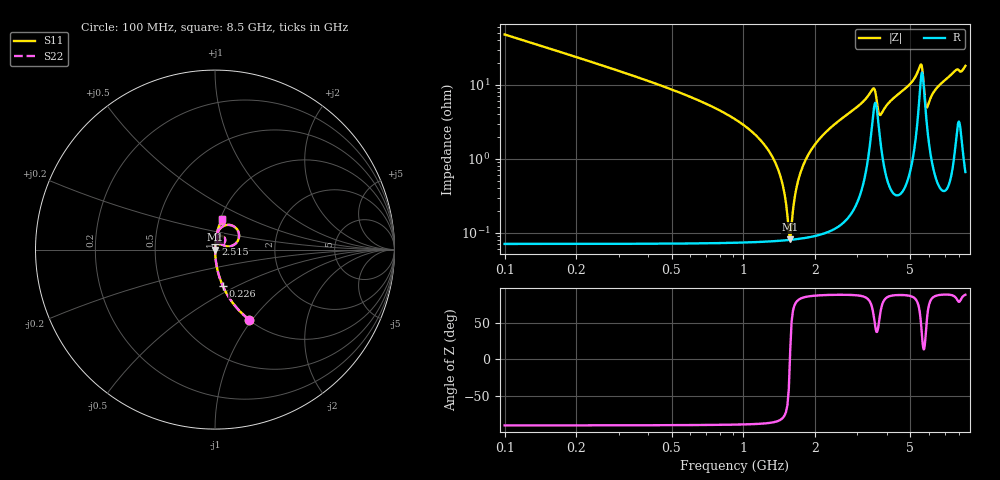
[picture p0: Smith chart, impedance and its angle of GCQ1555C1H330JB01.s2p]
!Murata Part Number: GCQ1555C1H330JB01
!These Parameters are Measured in Series Mode Connection
!Data Generated on Mar 13, 2026
!  o--ll--o
!Port1  Port2
!  o------o
!Operation Temp=25[degC], DC Bias Voltage=0[V]
!Freq. Start=100[MHz] Stop=9[GHz] 401[Steps]
# Hz S RI R 50
!Freq.(Hz) S11(Real) S11(Imag) S21(Real) S21(Imag) S12(Real) S12(Imag) S22(Real) S22(Imag)
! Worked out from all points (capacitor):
!   401 points, 100 MHz to 8.5 GHz, reference 50 ohm
!   read as one part in series: C = 33 pF near 142 MHz
!   lowest |Z| = 82.3 mohm at 1.57 GHz (marker M1)
!   series resonance near 1.566 GHz, so ESL is about 310 pH
!   S11 on the Smith chart (normalised r, x): 100 MHz: 1.00, -0.96; 226 MHz: 1.00, -0.42; 2.515 GHz: 1.00, +0.07; 8.5 GHz: 1.01, +0.36
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1e8  0.1878 -0.3898  0.8122 0.3898  0.8122 0.3898  0.1878 -0.3898
2.26e8  0.0425 -0.2  0.9575 0.2  0.9575 0.2  0.0425 -0.2
4.57e8  0.00996 -0.0957  0.99 0.0957  0.99 0.0957  0.00996 -0.0957
1.234e9  0.000986 -0.015  0.999 0.015  0.999 0.015  0.000986 -0.015
1.402e9  0.000829 -0.00693  0.9992 0.00693  0.9992 0.00693  0.000829 -0.00693
1.507e9  0.000801 -0.00241  0.9992 0.00241  0.9992 0.00241  0.000801 -0.00241
1.57e9  0.000805 0.000168  0.9992 -0.000168  0.9992 -0.000168  0.000805 0.000168
1.696e9  0.000854 0.00506  0.9991 -0.00506  0.9991 -0.00506  0.000854 0.00506
1.843e9  0.000971 0.0104  0.999 -0.0104  0.999 -0.0104  0.000971 0.0104
2.116e9  0.00134 0.0197  0.9987 -0.0197  0.9987 -0.0197  0.00134 0.0197
2.515e9  0.00231 0.0328  0.9977 -0.0328  0.9977 -0.0328  0.00231 0.0328
2.914e9  0.00433 0.0468  0.9957 -0.0468  0.9957 -0.0468  0.00433 0.0468
3.481e9  0.0402 0.0752  0.9598 -0.0752  0.9598 -0.0752  0.0402 0.0752
3.733e9  0.0197 0.033  0.9803 -0.033  0.9803 -0.033  0.0197 0.033
4.3e9  0.00789 0.0675  0.9921 -0.0675  0.9921 -0.0675  0.00789 0.0675
5.518e9  0.1139 0.1229  0.8861 -0.1229  0.8861 -0.1229  0.1139 0.1229
5.602e9  0.1327 0.0629  0.8673 -0.0629  0.8673 -0.0629  0.1327 0.0629
5.707e9  0.0782 0.0178  0.9218 -0.0178  0.9218 -0.0178  0.0782 0.0178
5.854e9  0.0311 0.0361  0.9689 -0.0361  0.9689 -0.0361  0.0311 0.0361
6.316e9  0.013 0.0816  0.987 -0.0816  0.987 -0.0816  0.013 0.0816
7.114e9  0.0185 0.1195  0.9815 -0.1195  0.9815 -0.1195  0.0185 0.1195
8.5e9  0.0376 0.1728  0.9624 -0.1728  0.9624 -0.1728  0.0376 0.1728
